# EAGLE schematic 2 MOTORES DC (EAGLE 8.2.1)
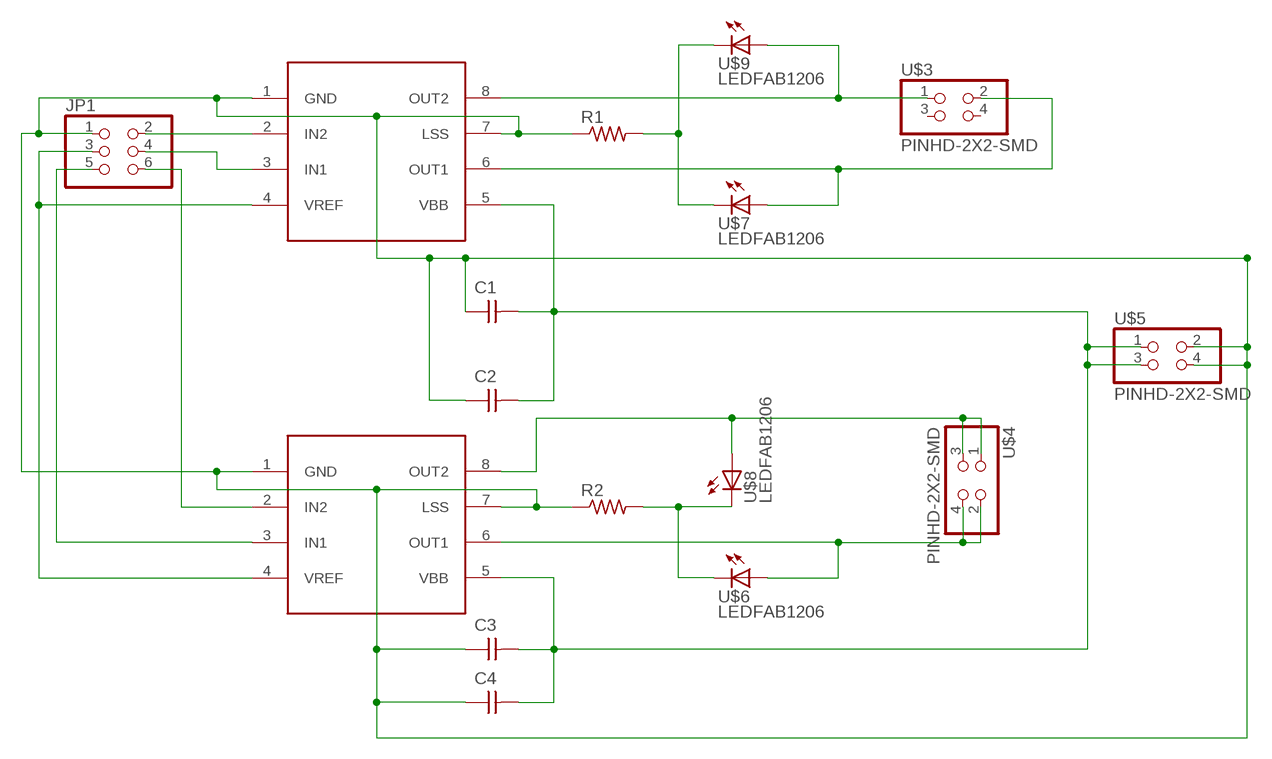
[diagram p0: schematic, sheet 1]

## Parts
C1  CAP-UNPOLARIZEDFAB  [C1206FAB]
C2  CAP-UNPOLARIZEDFAB  [C1206FAB]
C3  CAP-UNPOLARIZEDFAB  [C1206FAB]
C4  CAP-UNPOLARIZEDFAB  [C1206FAB]
JP1  PINHD-2X3-SMD  [2X03SMD]
R1  RES-US1206FAB  [R1206FAB]
R2  RES-US1206FAB  [R1206FAB]
U$1  A4953-H-BRIDGE-MOTOR-DRIVER  [SOIC8]
U$2  A4953-H-BRIDGE-MOTOR-DRIVER  [SOIC8]
U$3  PINHD-2X2-SMD  [2X02SMD]
U$4  PINHD-2X2-SMD  [2X02SMD]
U$5  PINHD-2X2-SMD  [2X02SMD]
U$6  LEDFAB1206  [LED1206FAB]
U$7  LEDFAB1206  [LED1206FAB]
U$8  LEDFAB1206  [LED1206FAB]
U$9  LEDFAB1206  [LED1206FAB]

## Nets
N$1: JP1.2 U$1.2(IN2)
N$2: JP1.4 U$1.3(IN1)
N$3: C1.2 C2.2 C3.2 C4.2 U$1.5(VBB) U$2.5(VBB) U$5.1 U$5.3
N$4: JP1.6 U$2.2(IN2)
N$5: JP1.5 U$2.3(IN1)
N$6: JP1.3 U$1.4(VREF) U$2.4(VREF)
N$7: U$1.8(OUT2) U$3.1 U$9.1(A)
N$8: U$1.6(OUT1) U$3.2 U$7.1(A)
N$9: U$2.8(OUT2) U$4.1 U$4.3 U$8.1(A)
N$10: U$2.6(OUT1) U$4.2 U$4.4 U$6.1(A)
N$12: C1.1 C2.1 C3.1 C4.1 JP1.1 R1.1 R2.1 U$1.1(GND) U$1.7(LSS) U$2.1(GND) U$2.7(LSS) U$5.2 U$5.4
N$13: R2.2 U$6.2(C) U$8.2(C)
N$14: R1.2 U$7.2(C) U$9.2(C)
Unconnected: U$3.3 U$3.4

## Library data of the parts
C1-C4 = fab (1):CAP-UNPOLARIZED
JP1 = fab (1):PINHD-2X3-SMD: PIN HEADER
R1 R2 = fab (1):RES-US: Resistor (US Symbol)
U$1 U$2 = fab (1):A4953-H-BRIDGE-MOTOR-DRIVER
U$3-U$5 = fab (1):PINHD-2X2-SMD
U$6-U$9 = fab (1):LED: LED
